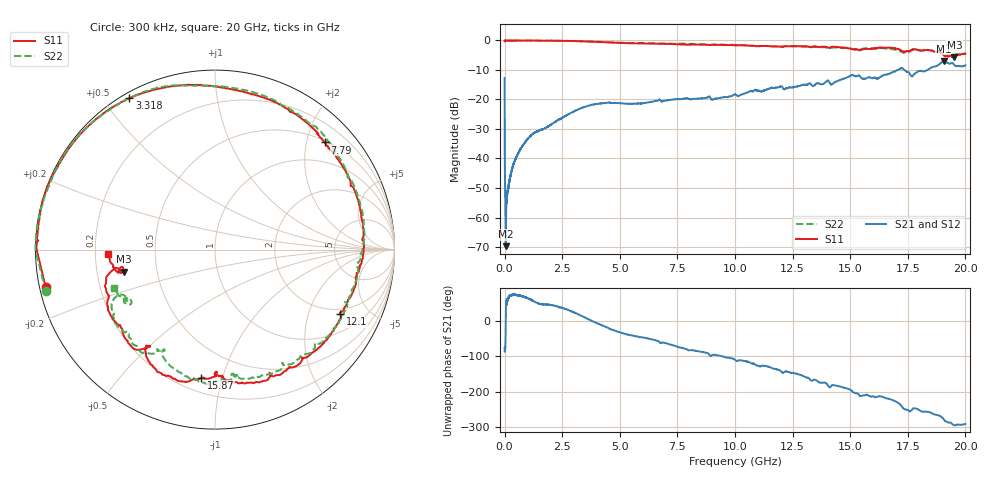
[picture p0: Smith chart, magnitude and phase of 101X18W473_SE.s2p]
!{101X18W473_SE}
!Johanson Technology Inc.
!www.johansontechnology.com
!Test Board Conditions:
!Substrate Type  RO4350B
!Substrate Thickness  21 mil
!Substrate Dk  3.66
!TL Type: GCPW
!TL Trace Width  40 mil
!TL Gap  20 mil
!PART MODE SINGLE ENDED (AKA BYPASS)
!DUT TOPOLOGY	SERIES-SHUNT
!Mounting Pad LxW  120x40 mil
! Created Wed Oct 27 11:09:09 2021
# hz S ma R 50
! 2 Port Network Data from SP1.SP block
! freq  magS11  angS11  magS21  angS21  magS12  angS12  magS22  angS22
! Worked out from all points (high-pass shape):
!   20001 points, 300 kHz to 20 GHz, reference 50 ohm
!   highest |S21| = -6.96 dB at 19.07 GHz (marker M1); lowest = -69.7 dB at 48.3 MHz (marker M2)
!   |S21| within 3 dB of the highest: 17.08 GHz to 17.34 GHz (262 MHz wide, 1.52 % of centre); 18.37 GHz to end of sweep
!   lowest |S11| = -5.7 dB at 19.52 GHz (marker M3), VSWR 3.17, Z = 16 - j5.36 ohm
!   |S11| at or under -10 dB: nowhere
!   |S22| runs from -5.3 to 0.0 dB; largest |S21 - S12| = 0.012
!   S11 on the Smith chart (normalised r, x): 300 kHz: 0.02, -0.11; 3.318 GHz: 0.02, +0.58; 7.79 GHz: 0.53, +2.35; 12.1 GHz: 1.75, -3.26; 15.87 GHz: 0.29, -0.86; 20 GHz: 0.25, -0.02
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300000  0.9664 -167.6  0.2317 -75.8  0.2325 -76.5  0.9712 -166.3
4.83e7  0.9936 179.2  0.000327 -26.9  0.0004168 -12.8  1 179.2
1.013e8  0.9938 178.2  0.002095 59.6  0.001968 59.7  0.9998 178.2
1.183e8  0.9947 177.8  0.002572 62.5  0.002615 62.3  0.9986 177.9
2.173e8  0.9935 176.0  0.004395 70.9  0.004454 70.9  0.9998 176.1
4.013e8  0.994 172.6  0.008236 74.3  0.008326 74.7  0.9997 172.8
9.733e8  0.9988 162.4  0.02072 66.1  0.0208 66.3  0.994 162.8
3.3183e9  0.9681 119.5  0.07104 15.8  0.07134 15.8  0.9705 120.3
3.3343e9  0.9674 119.2  0.07161 15.3  0.07169 15.3  0.9693 119.9
4.7593e9  0.9174 94.2  0.08725 -26.1  0.08766 -26.1  0.921 97.3
6.6673e9  0.8816 62.6  0.09663 -56.4  0.09681 -56.7  0.8927 66.3
7.7903e9  0.8545 44.3  0.1035 -77.3  0.1031 -77.0  0.8788 46.9
1.00003e10  0.8249 4.5  0.1222 -109.9  0.123 -109.8  0.8355 9.3
1.20983e10  0.7845 -27.2  0.1513 -146.7  0.1499 -146.6  0.7888 -21.8
1.33343e10  0.7795 -51.3  0.1751 -169.4  0.1759 -168.8  0.77 -43.7
1.43823e10  0.7756 -72.2  0.2007 177.3  0.2026 177.5  0.7594 -65.8
1.58683e10  0.7174 -96.1  0.2362 146.4  0.2366 146.0  0.7218 -87.1
1.66673e10  0.7538 -111.4  0.2708 139.6  0.2691 141.5  0.7274 -101.7
1.84033e10  0.6836 -149.3  0.3244 102.3  0.3248 102.0  0.6921 -143.5
1.90653e10  0.56 -169.5  0.4488 80.8  0.4474 81.0  0.5804 -154.4
1.95203e10  0.5206 -166.4  0.386 64.0  0.3842 63.9  0.5613 -147.1
2e10  0.5942 -177.7  0.3811 68.0  0.381 67.2  0.6001 -159.7
